(* Logix 5000 AddOnInstructionDefinition export i550ExplicitMSGHandler; software revision 20.00 *)

ADD_ON_INSTRUCTION i550ExplicitMSGHandler   (* revision 1.0 *)
// Parameterize i550.
VAR_INPUT
   xSend : BOOL;   // Send messages.
   diActivateNetworkControl : DINT := 1; {visible}   // P400:37 - Setting value [1] for Constant TRUE is required for network control.
   diEnableInverter : DINT := 1; {visible}   // P400:1 - Set value to [1] for Constant TRUE. This bypasses the need for a hardware enable signal.
   diRun : DINT := 1; {visible}   // P400:2 - Setting value [1] for Constant TRUE is recommended for network control.
   diSetpointSource : DINT := 5; {visible}   // P201:1 - Setting value [5] for Network is required for network control.
   diMainsVoltage : DINT; {visible}   // P208:1 - 230 V [0], 400 V [1], 480 V [2]
   diMotorRatedRPM : DINT := 1750; {visible}   // P320:4 - [RPM]
   rMotorRatedCurrent : REAL := 1.7; {visible}   // P323 - [Amps]
   rMotorRatedFrequency : REAL := 60.0; {visible}   // P320:5 - [Hz]
   rAccelTime : REAL := 5.0; {visible}   // P220 - Accel time [seconds]
   rDecelTime : REAL := 5.0; {visible}   // P221 - Decel time [seconds]
   rQspDecelTime : REAL := 1.0; {visible}   // P225 - Quickstop decel time [seconds]
END_VAR
VAR_OUTPUT
   Value_Out : DINT; {access Read Only}   // Value being sent to i550 parameter
   xDone : BOOL; {access Read Only, visible}   // All messages sent
END_VAR
VAR_IN_OUT
   MSG_Out : MESSAGE; {required}   // Reference to external MSG instruction
END_VAR
VAR
   iParameterCount : INT := 1; {access None}
   xOSR_out : BOOL; {access None}
   xOSR_storage : BOOL; {access None}
END_VAR

ROUTINE Logic   (* ladder *)
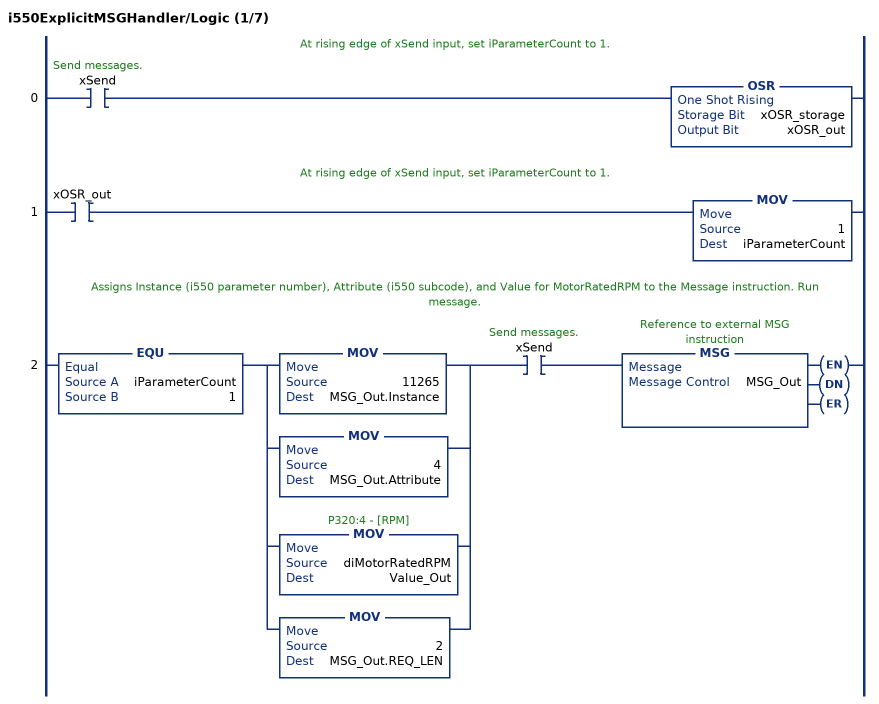
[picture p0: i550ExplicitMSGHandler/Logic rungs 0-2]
   // At rising edge of xSend input, set iParameterCount to 1.
   0: XIC(xSend)OSR(xOSR_storage,xOSR_out);
   // At rising edge of xSend input, set iParameterCount to 1.
   1: XIC(xOSR_out)MOV(1,iParameterCount);
   // Assigns Instance (i550 parameter number), Attribute (i550 subcode), and Value for MotorRatedRPM to the Message instruction. Run message.
   2: EQU(iParameterCount,1)[MOV(11265,MSG_Out.Instance) ,[MOV(4,MSG_Out.Attribute) ,MOV(diMotorRatedRPM,Value_Out) ,MOV(2,MSG_Out.REQ_LEN) ] ]XIC(xSend)MSG(MSG_Out);
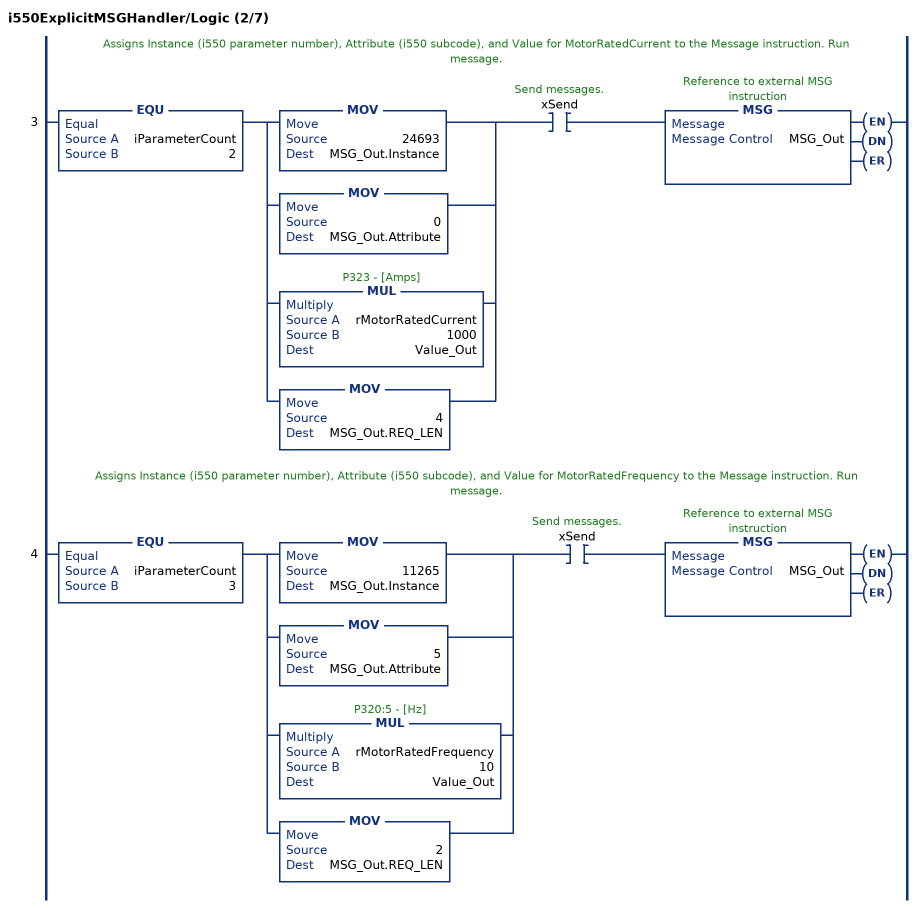
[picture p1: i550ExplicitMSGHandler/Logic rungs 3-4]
   // Assigns Instance (i550 parameter number), Attribute (i550 subcode), and Value for MotorRatedCurrent to the Message instruction. Run message.
   3: EQU(iParameterCount,2)[MOV(24693,MSG_Out.Instance) ,[MOV(0,MSG_Out.Attribute) ,MUL(rMotorRatedCurrent,1000,Value_Out) ,MOV(4,MSG_Out.REQ_LEN) ] ]XIC(xSend)MSG(MSG_Out);
   // Assigns Instance (i550 parameter number), Attribute (i550 subcode), and Value for MotorRatedFrequency to the Message instruction. Run message.
   4: EQU(iParameterCount,3)[MOV(11265,MSG_Out.Instance) ,[MOV(5,MSG_Out.Attribute) ,MUL(rMotorRatedFrequency,10,Value_Out) ,MOV(2,MSG_Out.REQ_LEN) ] ]XIC(xSend)MSG(MSG_Out);
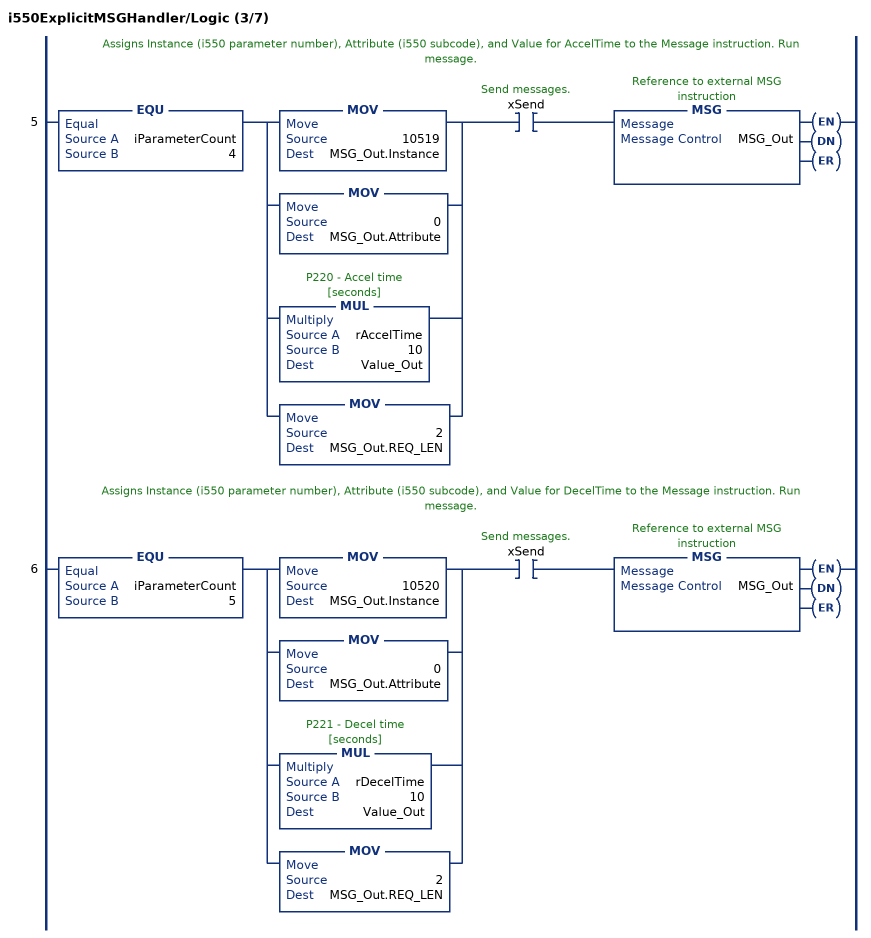
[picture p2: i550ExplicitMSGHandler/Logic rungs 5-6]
   // Assigns Instance (i550 parameter number), Attribute (i550 subcode), and Value for AccelTime to the Message instruction. Run message.
   5: EQU(iParameterCount,4)[MOV(10519,MSG_Out.Instance) ,[MOV(0,MSG_Out.Attribute) ,MUL(rAccelTime,10,Value_Out) ,MOV(2,MSG_Out.REQ_LEN) ] ]XIC(xSend)MSG(MSG_Out);
   // Assigns Instance (i550 parameter number), Attribute (i550 subcode), and Value for DecelTime to the Message instruction. Run message.
   6: EQU(iParameterCount,5)[MOV(10520,MSG_Out.Instance) ,[MOV(0,MSG_Out.Attribute) ,MUL(rDecelTime,10,Value_Out) ,MOV(2,MSG_Out.REQ_LEN) ] ]XIC(xSend)MSG(MSG_Out);
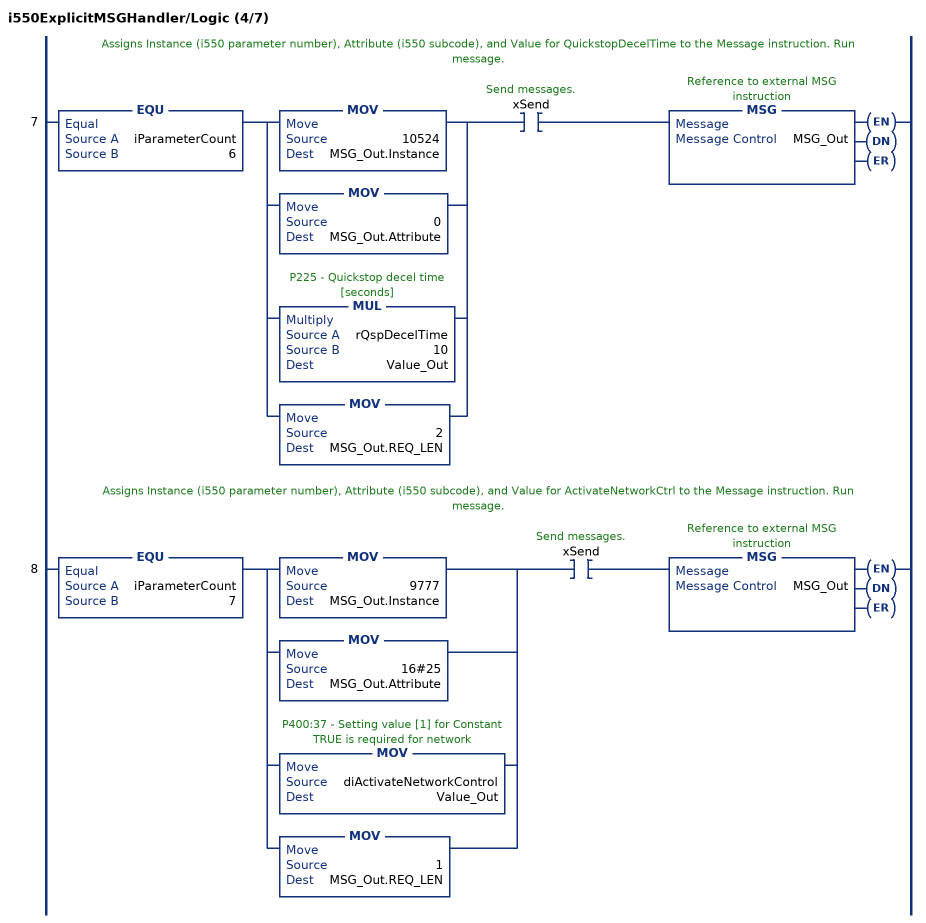
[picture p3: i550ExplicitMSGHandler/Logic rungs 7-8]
   // Assigns Instance (i550 parameter number), Attribute (i550 subcode), and Value for QuickstopDecelTime to the Message instruction. Run message.
   7: EQU(iParameterCount,6)[MOV(10524,MSG_Out.Instance) ,[MOV(0,MSG_Out.Attribute) ,MUL(rQspDecelTime,10,Value_Out) ,MOV(2,MSG_Out.REQ_LEN) ] ]XIC(xSend)MSG(MSG_Out);
   // Assigns Instance (i550 parameter number), Attribute (i550 subcode), and Value for ActivateNetworkCtrl to the Message instruction. Run message.
   8: EQU(iParameterCount,7)[MOV(9777,MSG_Out.Instance) ,[MOV(16#25,MSG_Out.Attribute) ,MOV(diActivateNetworkControl,Value_Out) ,MOV(1,MSG_Out.REQ_LEN) ] ]XIC(xSend)MSG(MSG_Out);
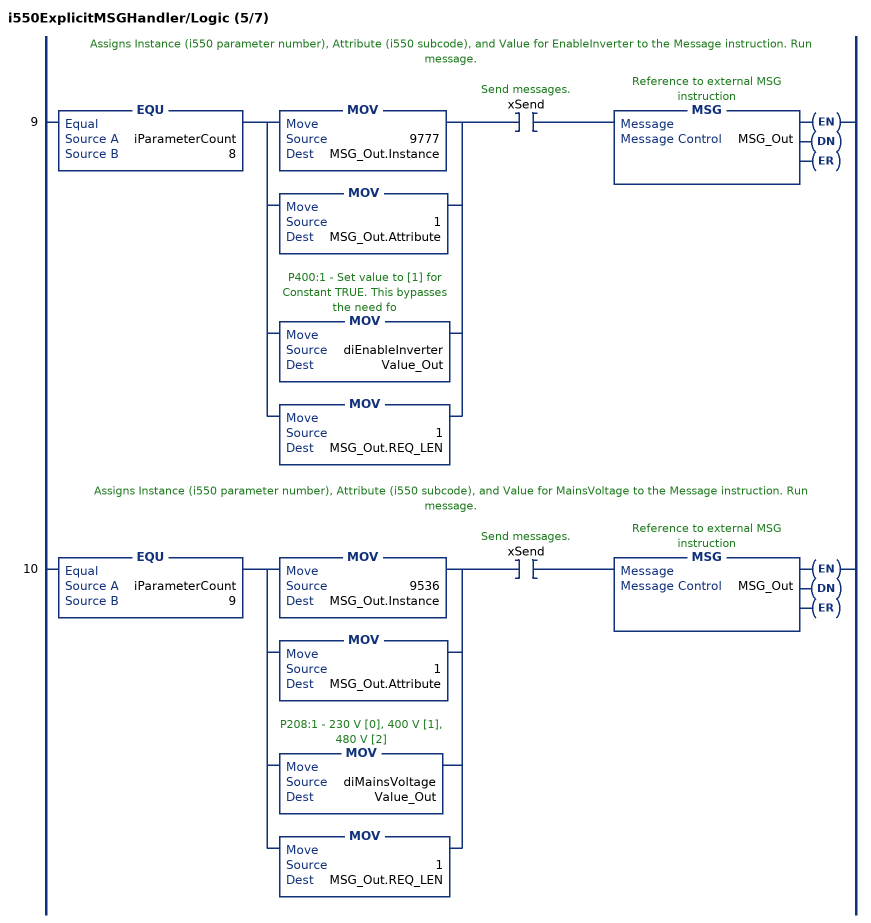
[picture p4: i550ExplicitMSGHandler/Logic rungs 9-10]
   // Assigns Instance (i550 parameter number), Attribute (i550 subcode), and Value for EnableInverter to the Message instruction. Run message.
   9: EQU(iParameterCount,8)[MOV(9777,MSG_Out.Instance) ,[MOV(1,MSG_Out.Attribute) ,MOV(diEnableInverter,Value_Out) ,MOV(1,MSG_Out.REQ_LEN) ] ]XIC(xSend)MSG(MSG_Out);
   // Assigns Instance (i550 parameter number), Attribute (i550 subcode), and Value for MainsVoltage to the Message instruction. Run message.
   10: EQU(iParameterCount,9)[MOV(9536,MSG_Out.Instance) ,[MOV(1,MSG_Out.Attribute) ,MOV(diMainsVoltage,Value_Out) ,MOV(1,MSG_Out.REQ_LEN) ] ]XIC(xSend)MSG(MSG_Out);
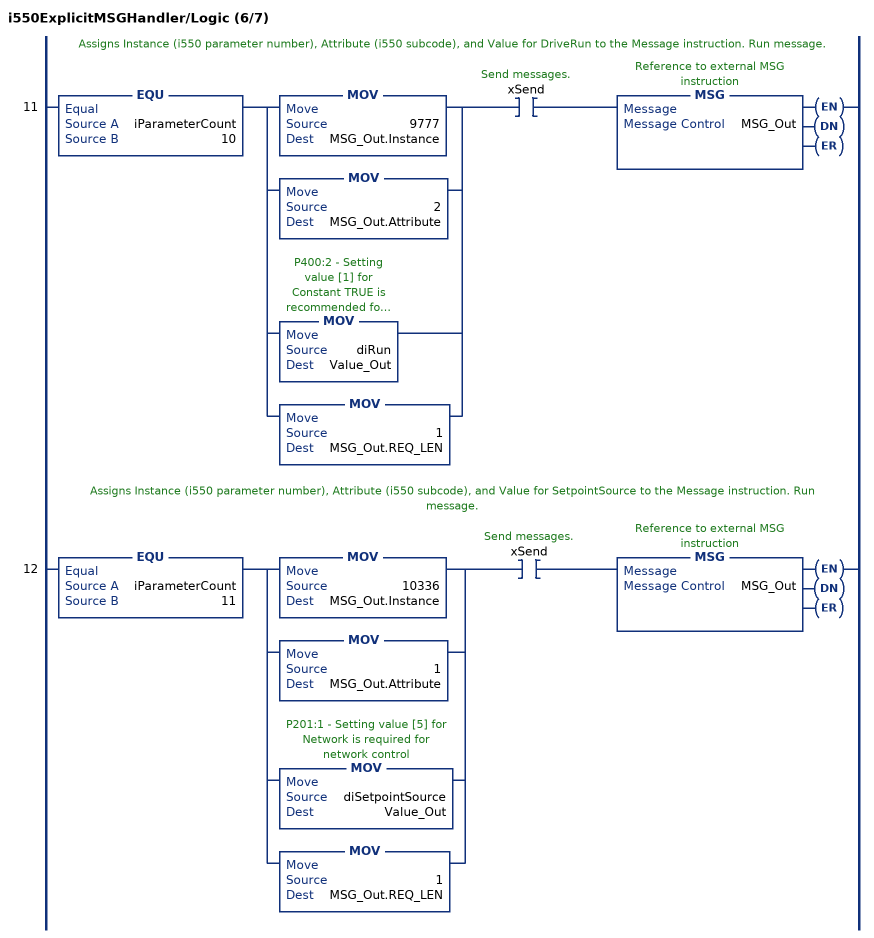
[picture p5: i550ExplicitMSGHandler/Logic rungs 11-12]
   // Assigns Instance (i550 parameter number), Attribute (i550 subcode), and Value for DriveRun to the Message instruction. Run message.
   11: EQU(iParameterCount,10)[MOV(9777,MSG_Out.Instance) ,[MOV(2,MSG_Out.Attribute) ,MOV(diRun,Value_Out) ,MOV(1,MSG_Out.REQ_LEN) ] ]XIC(xSend)MSG(MSG_Out);
   // Assigns Instance (i550 parameter number), Attribute (i550 subcode), and Value for SetpointSource to the Message instruction. Run message.
   12: EQU(iParameterCount,11)[MOV(10336,MSG_Out.Instance) ,[MOV(1,MSG_Out.Attribute) ,MOV(diSetpointSource,Value_Out) ,MOV(1,MSG_Out.REQ_LEN) ] ]XIC(xSend)MSG(MSG_Out);
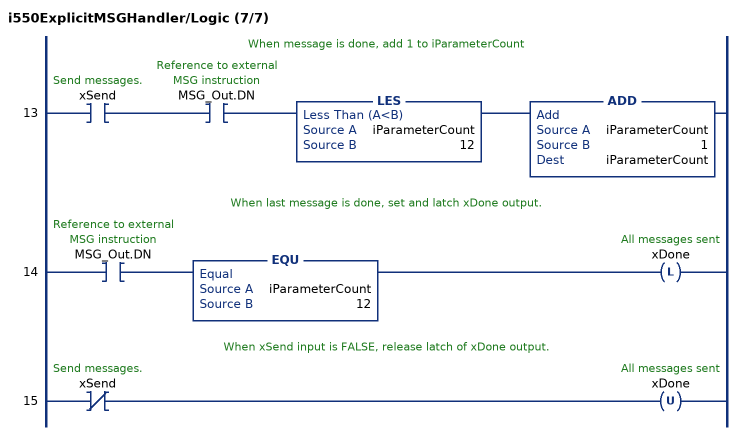
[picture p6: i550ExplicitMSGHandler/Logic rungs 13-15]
   // When message is done, add 1 to iParameterCount
   13: XIC(xSend)XIC(MSG_Out.DN)LES(iParameterCount,12)ADD(iParameterCount,1,iParameterCount);
   // When last message is done, set and latch xDone output.
   14: XIC(MSG_Out.DN)EQU(iParameterCount,12)OTL(xDone);
   // When xSend input is FALSE, release latch of xDone output.
   15: XIO(xSend)OTU(xDone);
END_ROUTINE
END_ADD_ON_INSTRUCTION
